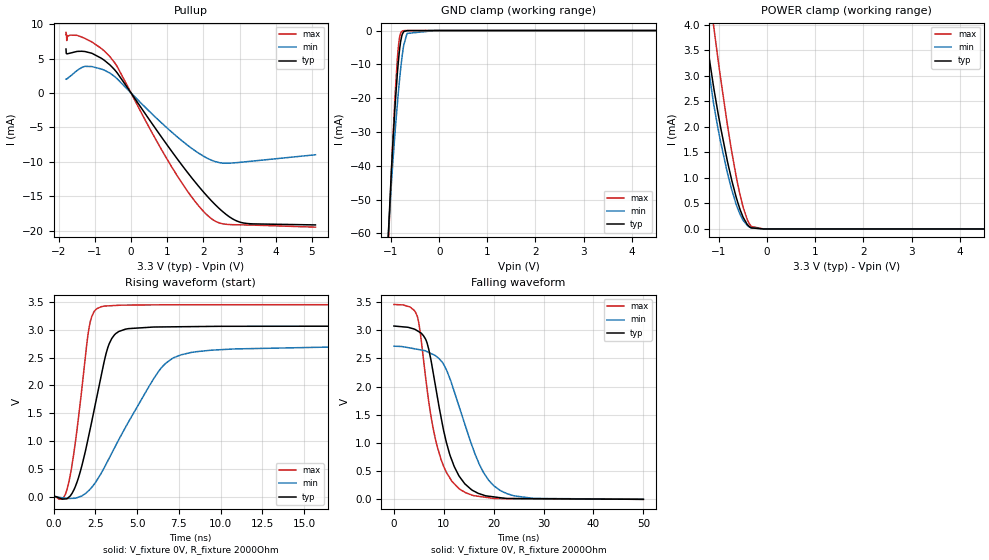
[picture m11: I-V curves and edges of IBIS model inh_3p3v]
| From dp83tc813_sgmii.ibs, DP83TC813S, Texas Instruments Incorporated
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| inh_3p3v
[Model]   inh_3p3v
Model_type   Open_source
Polarity   Non-Inverting
Vmeas = 1.65
Vref = 3.3
Cref = 2pF
Rref = 2000
|   typ   min   max
C_comp   1.30pF   1.27pF   1.33pF
[Voltage Range]   3.3   2.97   3.63
[Temperature Range]   27   150   -40
[Pullup Reference]   3.3   2.97   3.63
[Pulldown Reference]   0   0   0
[Power Clamp Reference]   3.3   2.97   3.63
[GND Clamp Reference]   0   0   0
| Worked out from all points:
|   slope of the pullup table from 0 to 0.495 V, typ, clamps not added: 130 ohm
|   GND clamp passes 1 mA (typ) near -0.76 V on its own axis
|   POWER clamp passes 1 mA (typ) near -0.75 V on its own axis
|   falling waveform, V_fixture 0V, R_fixture 2000Ohm: 20-80 % time 4.5ns typ, 6.48ns min, 3.97ns max; typ from 3.07 V to 0 V
|   rising waveform, V_fixture 0V, R_fixture 2000Ohm: 20-80 % time 1.31ns typ, 3.03ns min, 828ps max; typ from 0 V to 3.07 V
[GND Clamp]
|   Voltage   I(typ)   I(min)   I(max)
-1.8V     -305.2mA   -267.1mA   -333.8mA
-1.117V   -78.1mA    -74.4mA    -83.54mA
-992.7mV  -41.38mA   -45.14mA   -41.75mA
-923.7mV  -23.89mA   -31.31mA   -21.15mA
-861.6mV  -11.35mA   -20.42mA   -6.952mA
-840.9mV  -8.025mA   -17.12mA   -3.841mA
-820.2mV  -5.238mA   -14.02mA   -1.789mA
-771.9mV  -1.277mA   -7.742mA   -179.6uA
-737.4mV  -339.4uA   -4.348mA   -31.3uA
-668.4mV  -18.88uA   -857.9uA   -1.185uA
-68.1mV   0A         -6.227nA   0A
5.1V      0A         0A         0A
[Pullup]
|   Voltage   I(typ)   I(min)   I(max)
-1.8V     6.377mA    2.009mA    8.805mA
-1.786V   5.705mA    2.003mA    8.499mA
-1.779V   5.696mA    2.03mA     7.615mA
-1.772V   5.694mA    2.056mA    8.275mA
-1.676V   5.796mA    2.46mA     8.405mA
-1.276V   6.017mA    3.862mA    7.919mA
-461.4mV  3.408mA    2.414mA    4.448mA
1.139V    -8.587mA   -5.756mA   -10.87mA
1.774V    -12.95mA   -8.406mA   -15.79mA
2.23V     -15.7mA    -9.777mA   -18.29mA
3.023V    -18.78mA   -10.07mA   -19.15mA
5.1V      -19.16mA   -8.976mA   -19.49mA
[POWER Clamp]
|   Voltage   I(typ)   I(min)   I(max)
-1.8V     10.41mA    13.66mA    12.16mA
-1.31V    4.081mA    3.985mA    5.495mA
-1.227V   3.509mA    3.238mA    4.852mA
-1.103V   2.731mA    2.408mA    3.921mA
-972mV    2.022mA    1.734mA    2.991mA
-827.1mV  1.336mA    1.108mA    2.053mA
-647.7mV  638.6uA    497.5uA    1.056mA
-502.8mV  238.7uA    177.3uA    441uA
-371.7mV  46.46uA    39.16uA    103.6uA
-330.3mV  21.18uA    20.61uA    49.64uA
-68.1mV   0A         54.47nA    0A
5.1V      0A         0A         0A
[Ramp]
R_load = 2000
|   typ   min   max
dV/dt_r   1.84406/1.30667e-09   1.6295/3.02718e-09   2.07302/8.26905e-10
dV/dt_f   1.84404/4.48413e-09   1.6295/6.44583e-09   2.07303/3.95965e-09
[Falling Waveform]
V_fixture = 0V
V_fixture_min = 0V
V_fixture_max = 0V
R_fixture = 2000Ohm
C_fixture = 0F
|   Time   V(typ)   V(min)   V(max)
0s        3.073V     2.716V     3.455V
4.66ns    2.991V     2.661V     3.252V
6.4ns     2.83V      2.628V     2.128V
7.749ns   2.308V     2.573V     1.313V
9.449ns   1.455V     2.457V     707.4mV
11.1ns    823.1mV    2.169V     394.9mV
13.05ns   415.1mV    1.651V     189.9mV
17.21ns   96.89mV    604.3mV    50.33mV
21.51ns   26.47mV    147.4mV    13.56mV
50ns      2.349uV    0V         2.745uV
[Rising Waveform]
V_fixture = 0V
V_fixture_min = 0V
V_fixture_max = 0V
R_fixture = 2000Ohm
C_fixture = 0F
|   Time   V(typ)   V(min)   V(max)
0s        2.341uV    0V         2.571uV
877.4ps   -21.83mV   -35.46mV   208.7mV
1.423ns   273.5mV    -20.22mV   1.244V
2.133ns   1.13V      113.5mV    3.047V
2.871ns   2.199V     428.7mV    3.417V
3.336ns   2.752V     693mV      3.432V
3.907ns   2.97V      1.025V     3.441V
6.51ns    3.051V     2.335V     3.449V
8.31ns    3.057V     2.595V     3.45V
50ns      3.073V     2.716V     3.455V
